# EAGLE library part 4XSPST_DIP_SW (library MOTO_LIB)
4 channels SPST DIP switch 100mA.
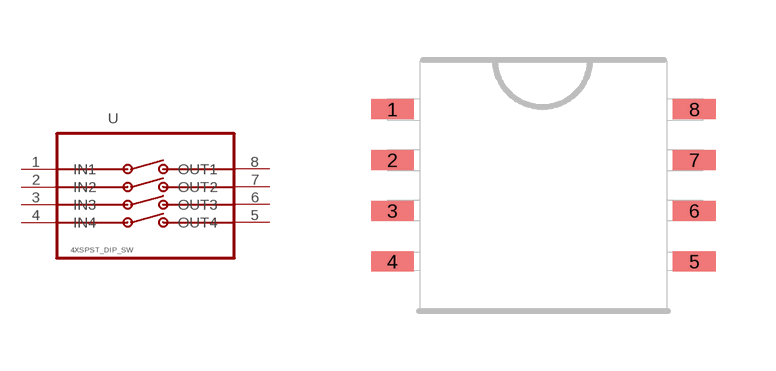
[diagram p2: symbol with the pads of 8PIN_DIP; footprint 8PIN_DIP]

Designator prefix U

## 4XSPST_DIP_SW (MPN: 1825140-2; SUPPLIER: TE CONNECTIVITY)  [8PIN_DIP]
1  IN1
2  IN2
3  IN3
4  IN4
5  OUT4
6  OUT3
7  OUT2
8  OUT1

## Footprint 8PIN_DIP (pad centres in mm)
DIP switch, 4 channel
smd 1.07 x 0.5: 1 -3.775,1.905; 2 -3.775,0.635; 3 -3.775,-0.636; 4 -3.775,-1.905; 5 3.775,-1.905; 6 3.775,-0.635; 7 3.775,0.635; 8 3.775,1.905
